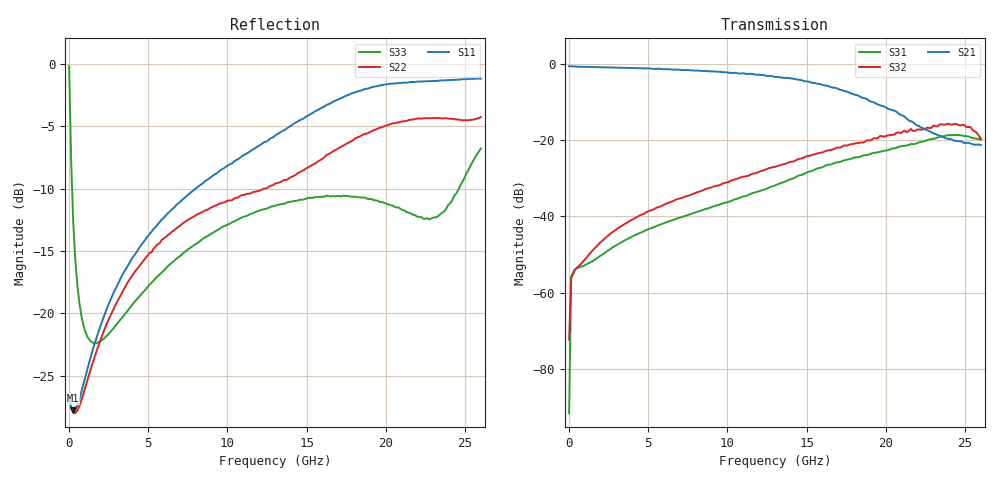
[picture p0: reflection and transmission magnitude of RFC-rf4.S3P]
!  3-Port S-parameters saved by WinCal
! VAR MeasName=S-Parameters (CALIBRATED_DATA) read from VNA (N5245A)
! VAR MeasDate=2016-7-4 10:43:25
! VAR NAME=25_C168105_RF1_RF4_11
! VAR FILENAME=25_C168105_RF1_RF4_11.S3P
! VAR DATE=2016-7-4 10:43:25
! VAR PHYS_PORTS=1,2,3
# Hz S DB R 50
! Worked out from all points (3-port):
!   201 points, 10 MHz to 26 GHz, reference 50 ohm
!   strongest paths, dB at 10 MHz, 6.508 GHz, 13.01 GHz, 19.5 GHz, 26 GHz:
!     S21: -0.6, -1.5, -3.4, -10.6, -21.3
!     S32: -72.4, -36.1, -27.0, -19.4, -19.6
!     S31: -91.7, -41.1, -31.9, -23.2, -19.8
!   lowest |S11| = -27.8 dB at 269.9 MHz (marker M1), VSWR 1.09, Z = 53.5 - j2.31 ohm
!   |S11| at or under -10 dB: start of sweep to 7.996 GHz
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1e7  -26.73 -3.3  -0.58 -0.3  -73.26 100.7
     -0.57 -0.3  -26.76 -4.8  -74.30 52.0
     -91.70 21.0  -72.37 43.7  -0.19 -9.3
1.3995e8  -27.53 -18.8  -0.62 -2.0  -55.63 41.2
          -0.61 -2.0  -27.61 -17.0  -56.15 43.7
          -55.84 41.3  -56.17 43.6  -7.78 -66.1
2.699e8  -27.78 -31.8  -0.66 -3.6  -54.72 29.4
         -0.65 -3.7  -27.94 -28.7  -55.03 36.0
         -54.68 28.5  -55.07 35.3  -12.70 -78.0
7.897e8  -26.27 -63.3  -0.74 -9.6  -53.14 27.0
         -0.74 -9.6  -26.96 -57.7  -52.30 41.2
         -53.13 27.5  -52.33 41.4  -20.25 -89.8
1.5694e9  -22.65 -88.1  -0.81 -18.3  -51.51 38.9
          -0.81 -18.4  -23.74 -81.7  -48.63 52.1
          -51.54 38.9  -48.63 52.1  -22.40 -96.9
6.7674e9  -11.33 -162.2  -1.47 -77.6  -40.69 42.3
          -1.44 -77.3  -13.21 -158.0  -35.61 25.1
          -40.64 42.5  -35.56 25.2  -15.65 -135.0
1.3005e10  -5.76 138.7  -3.47 -150.8  -32.03 18.7
           -3.40 -151.4  -9.61 94.9  -27.22 -35.3
           -31.88 17.9  -27.02 -35.2  -11.38 171.3
1.807305e10  -2.27 91.2  -8.61 141.3  -25.04 -29.8
             -8.09 143.9  -5.98 -22.6  -20.88 -100.1
             -24.51 -28.7  -20.82 -101.1  -10.65 116.2
2.145175e10  -1.48 58.7  -14.67 121.8  -21.29 -59.1
             -14.85 116.4  -4.50 -81.9  -17.63 -161.1
             -21.24 -62.2  -17.58 -159.0  -11.93 77.0
2.6e10  -1.18 22.5  -21.09 152.8  -19.90 -111.7
        -21.30 148.9  -4.27 -130.8  -19.81 92.4
        -19.83 -114.7  -19.57 93.9  -6.79 41.4
